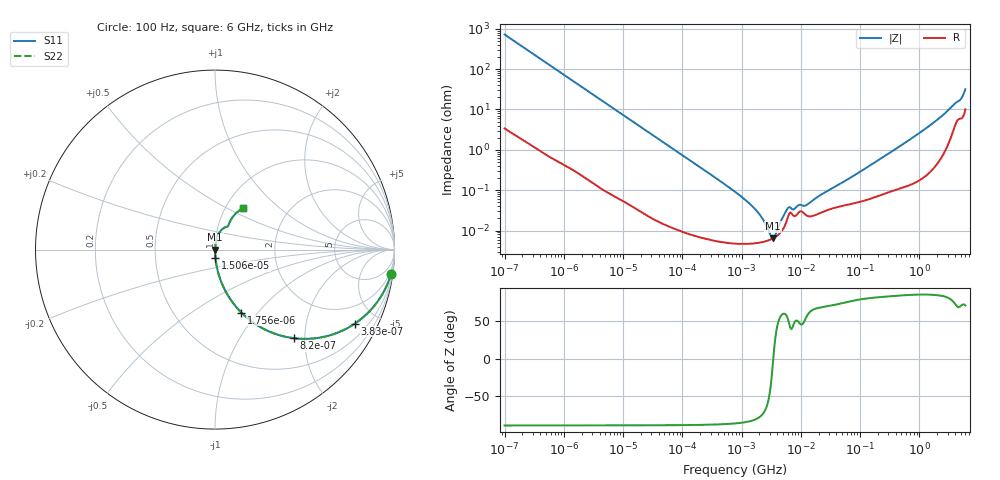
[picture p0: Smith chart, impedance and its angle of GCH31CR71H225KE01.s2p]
!Murata Part Number: GCH31CR71H225KE01
!These Parameters are Measured in Series Mode Connection
!Data Generated on Jun 19, 2026
!  o--ll--o
!Port1  Port2
!  o------o
!Operation Temp=25[degC], DC Bias Voltage=0[V]
!Freq. Start=100[Hz] Stop=6[GHz] 401[Steps]
# Hz S RI R 50
!Freq.(Hz) S11(Real) S11(Imag) S21(Real) S21(Imag) S12(Real) S12(Imag) S22(Real) S22(Imag)
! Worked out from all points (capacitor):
!   401 points, 100 Hz to 6 GHz, reference 50 ohm
!   read as one part in series: C = 2.21 uF near 109 Hz
!   lowest |Z| = 6.44 mohm at 3.394 MHz (marker M1)
!   series resonance near 3.429 MHz, so ESL is about 970 pH
!   S11 on the Smith chart (normalised r, x): 100 Hz: 1, -14; 383 Hz: 1.02, -3.77; 820 Hz: 1.01, -1.76; 1.756 kHz: 1.01, -0.83; 15.06 kHz: 1.00, -0.10; 6 GHz: 1.20, +0.60
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100  0.9804 -0.1363  0.0196 0.1363  0.0196 0.1363  0.9804 -0.1363
205  0.9242 -0.2622  0.0758 0.2622  0.0758 0.2622  0.9242 -0.2622
383  0.7791 -0.4123  0.2209 0.4123  0.2209 0.4123  0.7791 -0.4123
820  0.4381 -0.4934  0.5619 0.4934  0.5619 0.4934  0.4381 -0.4934
1756  0.1476 -0.3515  0.8524 0.3515  0.8524 0.3515  0.1476 -0.3515
2008  0.1173 -0.3186  0.8827 0.3186  0.8827 0.3186  0.1173 -0.3186
5143  0.0206 -0.1387  0.9794 0.1387  0.9794 0.1387  0.0206 -0.1387
15062  0.00273 -0.0485  0.9973 0.0485  0.9973 0.0485  0.00273 -0.0485
40335  0.000495 -0.0182  0.9995 0.0182  0.9995 0.0182  0.000495 -0.0182
774597  4.82e-05 -0.000914  1 0.000914  1 0.000914  4.82e-05 -0.000914
1585629  4.81e-05 -0.000373  1 0.000373  1 0.000373  4.81e-05 -0.000373
2074311  5.07e-05 -0.000231  0.9999 0.000231  0.9999 0.000231  5.07e-05 -0.000231
2837864  5.72e-05 -8.51e-05  0.9999 8.51e-05  0.9999 8.51e-05  5.72e-05 -8.51e-05
3394479  6.42e-05 -4.5e-06  0.9999 4.5e-06  0.9999 4.5e-06  6.42e-05 -4.5e-06
4060267  7.63e-05 7.91e-05  0.9999 -7.91e-05  0.9999 -7.91e-05  7.63e-05 7.91e-05
6075234  0.000218 0.000289  0.9998 -0.000289  0.9998 -0.000289  0.000218 0.000289
1.189169e7  0.000249 0.000331  0.9998 -0.000331  0.9998 -0.000331  0.000249 0.000331
1.555665e7  0.000229 0.000495  0.9998 -0.000495  0.9998 -0.000495  0.000229 0.000495
3.124326e8  0.000968 0.00825  0.999 -0.00825  0.999 -0.00825  0.000968 0.00825
2.048624e9  0.00779 0.0558  0.9922 -0.0558  0.9922 -0.0558  0.00779 0.0558
4.796499e9  0.0758 0.1375  0.9242 -0.1375  0.9242 -0.1375  0.0758 0.1375
6e9  0.1549 0.2317  0.8451 -0.2317  0.8451 -0.2317  0.1549 0.2317
